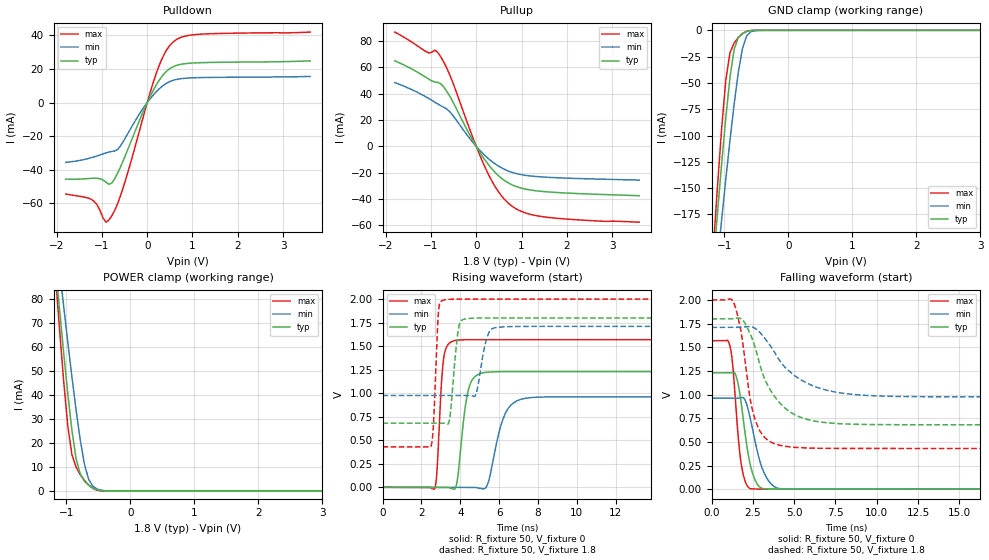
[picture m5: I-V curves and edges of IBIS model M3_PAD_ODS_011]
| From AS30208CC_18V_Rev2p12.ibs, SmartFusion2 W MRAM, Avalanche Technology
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[Model] M3_PAD_ODS_011
Model_type I/O
Enable   Active-High
Vinl  =  0.63
Vinh  =  1.17
Vmeas =  0.9
Cref  =  30e-12
| Capacitance  typ   min   max
C_comp   1.627116e-12   1.521588e-12   1.744735e-12
| Variables   typ   min   max
[GND Clamp Reference]   0   0   0
[POWER Clamp Reference]   1.8   1.71   2
[Pulldown Reference]   0   0   0
[Pullup Reference]   1.8   1.71   2
[Temperature Range]   25   125   -40
[Voltage Range]   1.8   1.71   2
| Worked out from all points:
|   slope of the pulldown table from 0 to 0.27 V, typ, clamps not added: 20 ohm
|   slope of the pullup table from 0 to 0.27 V, typ, clamps not added: 19.4 ohm
|   GND clamp passes 1 mA (typ) near -0.64 V on its own axis
|   POWER clamp passes 1 mA (typ) near -0.57 V on its own axis
|   falling waveform, R_fixture 50, V_fixture 0: 20-80 % time 624ps typ, 819ps min, 446ps max; typ from 1.23 V to 0 V
|   falling waveform, R_fixture 50, V_fixture 1.8: 20-80 % time 1.67ns typ, 2.39ns min, 857ps max; typ from 1.8 V to 0.681 V
|   rising waveform, R_fixture 50, V_fixture 0: 20-80 % time 415ps typ, 686ps min, 244ps max; typ from 0 V to 1.23 V
|   rising waveform, R_fixture 50, V_fixture 1.8: 20-80 % time 287ps typ, 388ps min, 188ps max; typ from 0.681 V to 1.8 V
[GND Clamp]
| Voltage   I(typ)   I(min)   I(max)
-1.8V     -720.5mA   -670.5mA   -825.4mA
-1.173V   -222.3mA   -260.3mA   -207.7mA
-1.108V   -173.8mA   -219.8mA   -148.5mA
-1.043V   -127mA     -180.1mA   -93.3mA
-977.6mV  -83.06mA   -141.5mA   -47.19mA
-912.4mV  -44.72mA   -104.6mA   -21.23mA
-847.2mV  -17.99mA   -70.1mA    -11.92mA
-782.1mV  -6.766mA   -39.85mA   -6.657mA
-716.9mV  -2.938mA   -17.13mA   -3.048mA
-651.7mV  -1.119mA   -5.25mA    -952uA
-456.2mV  -3.98uA    -74.41uA   -422.2nA
3.6V      0A         0A         0A
[POWER Clamp]
| Voltage   I(typ)   I(min)   I(max)
-1.8V     287.1mA    268.3mA    329.6mA
-1.173V   94.89mA    108.5mA    91.02mA
-1.108V   76.1mA     92.66mA    67.97mA
-1.043V   57.9mA     77.16mA    46.14mA
-977.6mV  40.62mA    62.05mA    27.14mA
-912.4mV  25.13mA    47.46mA    15.06mA
-847.2mV  13.38mA    33.64mA    9.853mA
-716.9mV  4.014mA    11.09mA    4.394mA
-651.7mV  2.34mA     4.821mA    2.483mA
-586.6mV  1.18mA     2.003mA    1.113mA
-325.9mV  1.153uA    19.85uA    110.1nA
3.6V      0A         0A         0A
[Pulldown]
| Voltage   I(typ)   I(min)   I(max)
-1.8V     -45.6mA    -35.58mA   -54.5mA
-1.238V   -45.15mA   -32.86mA   -57.63mA
-912.4mV  -47.36mA   -29.97mA   -71.26mA
-847.2mV  -48.69mA   -29.47mA   -70.02mA
-716.9mV  -45.3mA    -28.85mA   -64.14mA
-521.4mV  -34.03mA   -22.82mA   -49.79mA
-65.17mV  -3.915mA   -2.451mA   -6.278mA
248.3mV   12.65mA    7.772mA    20.97mA
434.5mV   18.83mA    11.62mA    31.58mA
620.7mV   21.87mA    13.59mA    37.09mA
1.179V    23.74mA    14.86mA    40.71mA
3.6V      24.84mA    15.54mA    41.96mA
[Pullup]
| Voltage   I(typ)   I(min)   I(max)
-1.8V     65.06mA    48.5mA     86.9mA
-1.108V   52.41mA    37.58mA    72.02mA
-912.4mV  48.87mA    33.57mA    73.19mA
-782.1mV  47.53mA    30.9mA     68.01mA
-521.4mV  34.19mA    23.72mA    48.98mA
-130.3mV  7.935mA    5.437mA    11.79mA
186.2mV   -9.992mA   -6.708mA   -15.2mA
496.6mV   -22.46mA   -15.07mA   -34.77mA
744.8mV   -28.41mA   -19.17mA   -44.22mA
1.055V    -32.21mA   -21.83mA   -50.2mA
1.49V     -34.31mA   -23.3mA    -53.53mA
3.6V      -37.46mA   -25.6mA    -57.6mA
[Ramp]
dV/dt_r   0.737574/0.415184n  0.576865/0.686423n  0.941389/0.244315n
dV/dt_f   0.671438/1.67409n  0.440569/2.39388n  0.941875/0.857114n
R_load = 50
[Falling Waveform]
R_fixture = 50
V_fixture = 0
V_fixture_min = 0
V_fixture_max = 0
| Time   V(typ)   V(min)   V(max)
0s        1.229V     961.4mV    1.569V
1.115ns   1.23V      961.9mV    1.511V
1.285ns   1.235V     962mV      1.306V
1.47ns    1.204V     962mV      876.8mV
1.778ns   933.2mV    966.6mV    285.8mV
2.293ns   299.1mV    786.5mV    9.213mV
2.659ns   86.73mV    485.6mV    1.715mV
3.073ns   7.118mV    218.5mV    941uV
4.053ns   960.7uV    7.909mV    188.7uV
21.88ns   -4.295nV   2.433uV    486.4nV
[Falling Waveform]
R_fixture = 50
V_fixture = 1.8
V_fixture_min = 1.71
V_fixture_max = 2
| Time   V(typ)   V(min)   V(max)
0s        1.8V       1.71V      2V
1.351ns   1.803V     1.71V      1.967V
1.767ns   1.804V     1.711V     1.684V
2.279ns   1.665V     1.718V     1.018V
2.532ns   1.556V     1.71V      796.9mV
3.067ns   1.237V     1.629V     576.6mV
3.843ns   972.7mV    1.438V     478.4mV
5.406ns   759.3mV    1.156V     438.3mV
7.716ns   692.4mV    1.02V      430.8mV
21.88ns   680.9mV    975.7mV    430.2mV
[Rising Waveform]
R_fixture = 50
V_fixture = 0
V_fixture_min = 0
V_fixture_max = 0
| Time   V(typ)   V(min)   V(max)
0s        1.871nV    42.98nV    67.84nV
2.689ns   -414uV     -306.8uV   -13.28mV
3.137ns   -482.9uV   -357.9uV   1.359V
3.61ns    -16.63mV   -411.9uV   1.553V
3.853ns   83.05mV    -439.6uV   1.563V
4.396ns   1.019V     -501.6uV   1.568V
5.002ns   1.207V     -10.54mV   1.568V
6.308ns   1.229V     779.8mV    1.568V
7.13ns    1.229V     935.5mV    1.568V
21.88ns   1.229V     961.4mV    1.569V
[Rising Waveform]
R_fixture = 50
V_fixture = 1.8
V_fixture_min = 1.71
V_fixture_max = 2
| Time   V(typ)   V(min)   V(max)
0s        680.9mV    975.7mV    430.2mV
2.495ns   681.6mV    976.2mV    436.7mV
2.872ns   681.7mV    976.3mV    1.854V
3.117ns   681.8mV    976.3mV    1.988V
3.448ns   721mV      976.4mV    1.998V
3.888ns   1.665V     976.5mV    1.999V
4.155ns   1.783V     976.5mV    1.999V
4.795ns   1.798V     982.7mV    1.999V
5.786ns   1.799V     1.695V     1.999V
21.88ns   1.8V       1.71V      2V
